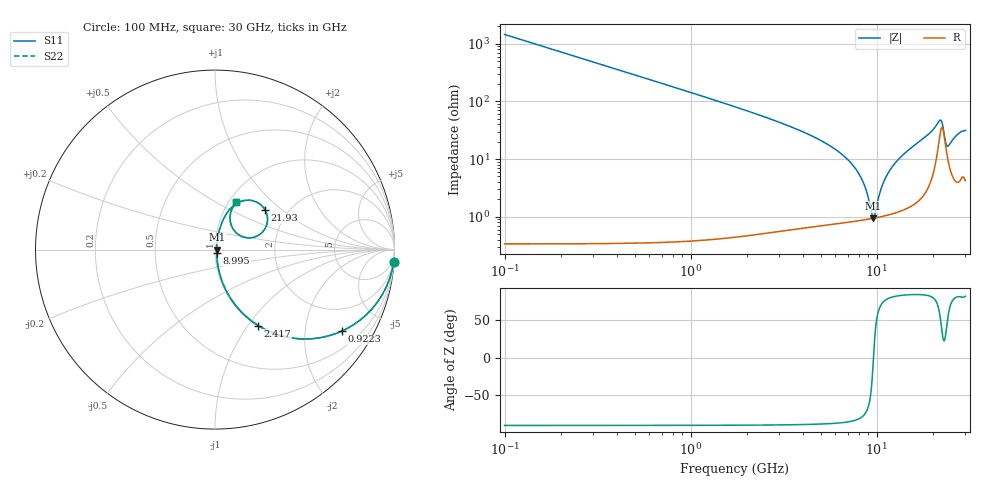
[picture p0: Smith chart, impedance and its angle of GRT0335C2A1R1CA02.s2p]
!Murata Part Number: GRT0335C2A1R1CA02
!These Parameters are Measured in Series Mode Connection
!Data Generated on Jun 19, 2026
!  o--ll--o
!Port1  Port2
!  o------o
!Operation Temp=25[degC], DC Bias Voltage=0[V]
!Freq. Start=100[MHz] Stop=30[GHz] 401[Steps]
# Hz S RI R 50
!Freq.(Hz) S11(Real) S11(Imag) S21(Real) S21(Imag) S12(Real) S12(Imag) S22(Real) S22(Imag)
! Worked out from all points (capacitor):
!   401 points, 100 MHz to 30 GHz, reference 50 ohm
!   read as one part in series: C = 1.1 pF near 249.5 MHz
!   lowest |Z| = 945 mohm at 9.593 GHz (marker M1)
!   series resonance near 9.616 GHz, so ESL is about 250 pH
!   S11 on the Smith chart (normalised r, x): 100 MHz: 1, -29; 922.2 MHz: 1.01, -3.11; 2.417 GHz: 1.01, -1.12; 8.995 GHz: 1.02, -0.04; 21.93 GHz: 1.54, +0.78; 30 GHz: 1.08, +0.62
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1e8  0.9952 -0.0688  0.00477 0.0688  0.00477 0.0688  0.9952 -0.0688
4.7375e8  0.9024 -0.2961  0.0976 0.2961  0.0976 0.2961  0.9024 -0.2961
9.2225e8  0.7066 -0.4541  0.2934 0.4541  0.2934 0.4541  0.7066 -0.4541
1.66975e9  0.4137 -0.4899  0.5863 0.4899  0.5863 0.4899  0.4137 -0.4899
2.41725e9  0.2405 -0.4229  0.7595 0.4229  0.7595 0.4229  0.2405 -0.4229
5.10825e9  0.0458 -0.1925  0.9542 0.1925  0.9542 0.1925  0.0458 -0.1925
7.64975e9  0.013 -0.0683  0.987 0.0683  0.987 0.0683  0.013 -0.0683
8.39725e9  0.0103 -0.0404  0.9897 0.0404  0.9897 0.0404  0.0103 -0.0404
8.99525e9  0.00939 -0.0199  0.9906 0.0199  0.9906 0.0199  0.00939 -0.0199
9.59325e9  0.00933 -0.000707  0.9907 0.000707  0.9907 0.000707  0.00933 -0.000707
9.74275e9  0.00944 0.00392  0.9906 -0.00392  0.9906 -0.00392  0.00944 0.00392
1.01165e10  0.00988 0.0152  0.9901 -0.0152  0.9901 -0.0152  0.00988 0.0152
1.078925e10  0.0113 0.0347  0.9887 -0.0347  0.9887 -0.0347  0.0113 0.0347
1.1761e10  0.0146 0.0611  0.9854 -0.0611  0.9854 -0.0611  0.0146 0.0611
1.505e10  0.0352 0.1414  0.9648 -0.1414  0.9648 -0.1414  0.0352 0.1414
2.005825e10  0.1297 0.2621  0.8703 -0.2621  0.8703 -0.2621  0.1297 0.2621
2.1927e10  0.2793 0.2208  0.7207 -0.2208  0.7207 -0.2208  0.2793 0.2208
2.289875e10  0.2328 0.0751  0.7672 -0.0751  0.7672 -0.0751  0.2328 0.0751
2.3721e10  0.1293 0.0848  0.8707 -0.0848  0.8707 -0.0848  0.1293 0.0848
2.50665e10  0.0846 0.1602  0.9154 -0.1602  0.9154 -0.1602  0.0846 0.1602
2.74585e10  0.0997 0.2354  0.9003 -0.2354  0.9003 -0.2354  0.0997 0.2354
3e10  0.119 0.2632  0.881 -0.2632  0.881 -0.2632  0.119 0.2632
